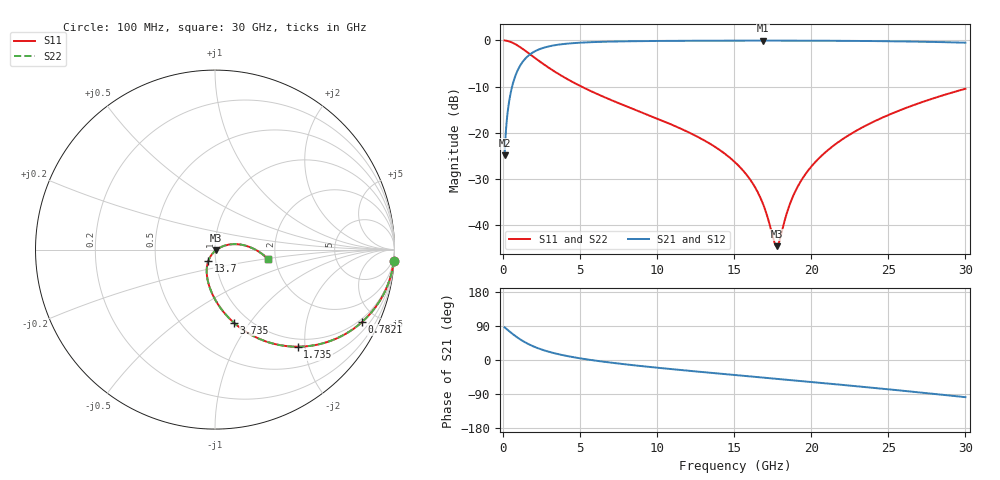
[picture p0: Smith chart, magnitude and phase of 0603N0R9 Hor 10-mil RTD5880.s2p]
# GHz S MA R 50
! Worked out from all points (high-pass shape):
!   3201 points, 100 MHz to 30 GHz, reference 50 ohm
!   highest |S21| = -0.05 dB at 16.85 GHz (marker M1); lowest = -24.9 dB at 100 MHz (marker M2)
!   |S21| within 3 dB of the highest: 1.74 GHz to end of sweep
!   lowest |S11| = -44.6 dB at 17.75 GHz (marker M3), VSWR 1.01, Z = 50.4 - j0.464 ohm
!   |S11| at or under -10 dB: 5.085 GHz to end of sweep
!   |S22| runs from -44.6 to 0.0 dB; largest |S21 - S12| = 0
!   S11 on the Smith chart (normalised r, x): 100 MHz: 1, -32; 782.1 MHz: 0.85, -4.13; 1.735 GHz: 0.85, -1.85; 3.735 GHz: 0.85, -0.84; 13.7 GHz: 0.92, -0.11; 30 GHz: 1.82, -0.21
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0.1  0.9982 -3.6  0.05694 86.3  0.05694 86.3  0.9982 -3.6
0.4083438  0.9736 -14.2  0.2261 75.6  0.2261 75.6  0.9736 -14.2
0.7820938  0.9132 -26.2  0.4062 63.7  0.4062 63.7  0.9132 -26.2
1.22125  0.8205 -38.3  0.5704 51.6  0.5704 51.6  0.8205 -38.3
1.735156  0.7101 -49.6  0.7026 40.2  0.7026 40.2  0.7101 -49.6
2.632156  0.5518 -63.9  0.8322 25.9  0.8322 25.9  0.5518 -63.9
3.734719  0.4193 -75.7  0.9056 14.1  0.9056 14.1  0.4193 -75.7
5.089563  0.3159 -85.7  0.9461 3.8  0.9461 3.8  0.3159 -85.7
10.06978  0.1407 -109.0  0.986 -20.6  0.986 -20.6  0.1407 -109.0
13.7045  0.07117 -120.8  0.9925 -34.7  0.9925 -34.7  0.07117 -120.8
15.05  0.04794 -123.5  0.9935 -39.7  0.9935 -39.7  0.04794 -123.5
16.0965  0.03002 -123.1  0.9939 -43.6  0.9939 -43.6  0.03002 -123.1
16.85334  0.01719 -117.1  0.994 -46.4  0.994 -46.4  0.01719 -117.1
17.57281  0.00676 -79.0  0.9939 -49.0  0.9939 -49.0  0.00676 -79.0
17.75034  0.00591 -51.2  0.9938 -49.7  0.9938 -49.7  0.00591 -51.2
17.92788  0.006704 -23.0  0.9938 -50.3  0.9938 -50.3  0.006704 -23.0
18.43244  0.01379 11.6  0.9936 -52.2  0.9936 -52.2  0.01379 11.6
18.85291  0.02119 19.2  0.9933 -53.8  0.9933 -53.8  0.02119 19.2
20.03956  0.04376 23.2  0.9922 -58.2  0.9922 -58.2  0.04376 23.2
22.06716  0.08596 19.3  0.9888 -65.9  0.9888 -65.9  0.08596 19.3
25.01978  0.156 9.6  0.9793 -77.4  0.9793 -77.4  0.156 9.6
30  0.2994 -10.0  0.9438 -98.1  0.9438 -98.1  0.2994 -10.0
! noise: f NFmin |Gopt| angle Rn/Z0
0.1  0.002978  0.9917  0.323  0.08264
3.417  0.004152  0.8153  10.44  0.004659
6.743  0.006818  0.7827  19.75  0.006254
10.06  0.009298  0.7664  28.97  0.007595
13.39  0.01171  0.7572  38.07  0.008741
16.7  0.01414  0.7527  46.93  0.009742
20.03  0.01664  0.7517  55.58  0.01063
23.35  0.01926  0.7535  63.96  0.01143
26.67  0.02207  0.7574  72.11  0.01215
30  0.02512  0.7632  80.01  0.0128
